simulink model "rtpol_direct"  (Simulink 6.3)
settings: Solver=ode45  SolverMode=SingleTasking  StartTime=0.0  StopTime=inf  FixedStep=h  RelTol=1e-3  AbsTol=1e-6
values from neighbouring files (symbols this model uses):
  adingain = [1.2*(pi*2/620/3)*[1 -1 -1 1 1 1] 1]    [hwinit.m]
  adinoffs = [-421 -511 -568 -518 -521 -410    0]    [hwinit.m]
  daoutgain = 127*[1 -1 -1 1 1 1 1]    [hwinit.m]
  daoutoffs = 127*[1 1 1 1 0.98 1 0]    [hwinit.m]
  h = 0.01    [design_pol.m]    (also in design_rot.m; design_wrist.m; rtrobot_init.m = 0.05; simpleregret.m = cfg.h)
  joint = [1 2 3 4 5]    [design_pol.m]    (also in design_rot.m = [1 5]; design_wrist.m = [5]; rtrobot_init.m = joint(:)+(0:6:6*(n-1))')
  Kd = [0.4 0.1 0.1]    [design_pol.m]    (also in design_rot.m = [0.3 0.1]; design_wrist.m = 0.01; mc_approx_vectorized.m = cfg.Kd)
  Ki = [0.6 0.3 0.9]/3    [design_pol.m]    (also in design_rot.m = [0.1 0.1]; design_wrist.m = 0)
  Kp = [0.5 0.2 1.0]    [design_pol.m]    (also in design_rot.m = [0.4 2]; design_wrist.m = 1.5)
undefined symbols (not defined in the file or in its folder): COM1, DiscIntNeverNeededParam, No
libraries: simulink x7, cstblocks x5, xpclib x4, rtlib x1

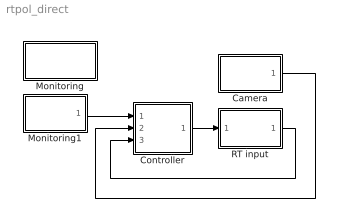
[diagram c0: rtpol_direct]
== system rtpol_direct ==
  Camera : Subsystem
  Controller : Subsystem
  Monitoring : Subsystem
  Monitoring1 : Subsystem
  RT input : Subsystem  InitFcn=rtclear all  mask{h=h, joint=joint, Port=COM1, laser=No, gripper=No}
      mask prompts: h "Sample time [s]:"; joint "Joints to control (e.g., [1 2 4])"; Port "Serial port:"; laser "Enable laser input"; gripper "Enable gripper current sensor"
      mask init:
      | hwinit;
      | sen = joint(:);                             % read joint angles
      | if strcmp(gripper,'Yes'),                   % if gripper current desired
      |     sen = [sen; 7];                         % add to the list
      | end;    
      |                                             
      | n = length(sen);                            % number of sensors to be read
      | sen = sen+(0:7:7*(n-1))';                   % convert into sequential index
      | sen_select = zeros(7,n);                    % prepare zeros
      | sen_select(sen) = 1;                        % assign 1 at the right places
      | 
      | act = joint(:);                             % control joint actuators
      | if strcmp(laser,'Yes'),                     % if laser desired
      |     act = [act; 7];                         % add to the list
      | end;    
      |                                             
      | n = length(act);                            % number of actuators to be controlled
      | act = act+(0:7:7*(n-1))';                   % convert into sequential index
      | act_select = zeros(7,n);                    % prepare zeros
      | act_select(act) = 1;                        % assign 1 at the right places
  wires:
  Camera/1(features) -> Controller/2(y)
  RT input/1(Angles) -> Controller/3(q)
  Monitoring1/1(r) -> Controller/1(r)
  Controller/1(out_2) -> RT input/1(Motors)

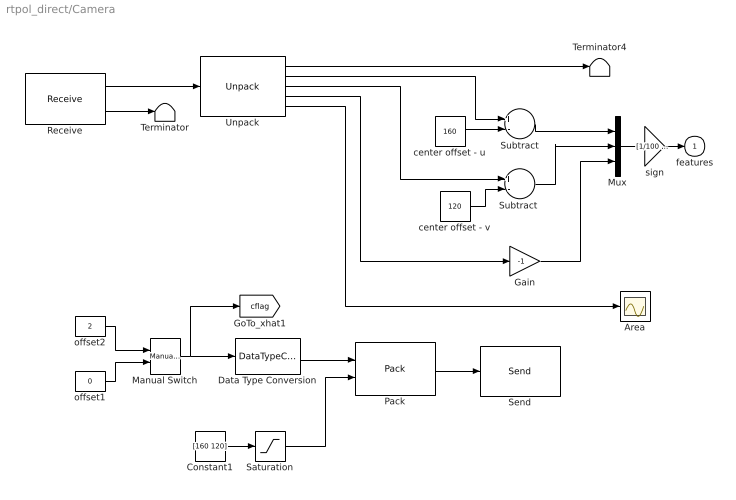
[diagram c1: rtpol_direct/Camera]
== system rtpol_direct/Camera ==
  Area : Scope
  Constant1 : Constant  Value=[160 120]
  Data Type Conversion : DataTypeConversion  OutDataTypeMode=uint8
  Gain : Gain  Gain=-1
  Manual Switch : simulink/Signal Routing/Manual Switch  sw=1  action=0
  Mux : Mux  Inputs=3
  Pack : xpclib/UDP/Pack  datatypes={'uint8','double'}  byteAlign=4
  Receive : xpclib/UDP/Receive  ipAddress=127.0.0.1  ipPort=6907  width=40  sampletime=h
  Saturation : Saturate  UpperLimit=[320 240]  LowerLimit=[0 0]
  Send : xpclib/UDP/Send  ipAddress=127.0.0.1  ipPort=6906  localPort=-1  sampletime=h
  Subtract : Sum  Inputs=+-  OutScaling=2^-10
  "Subtract " : Sum  Inputs=+-  OutScaling=2^-10
  Terminator : Terminator
  Terminator4 : Terminator
  Unpack : xpclib/UDP/Unpack  dimensions={1,1,1,1,1}  datatypes={'double','double','double','double','double'}  byteAlign=4
  center offset - u : Constant  Value=160
  center offset - v : Constant  Value=120
  offset1 : Constant  Value=0
  offset2 : Constant  Value=2
  sign : Gain  Gain=[1/100 1/100 1]  SampleTime=h
  features : Outport  InitialOutput=0
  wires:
  Receive/2 -> Terminator/1
  Receive/1 -> Unpack/1
  center offset - u/1 -> Subtract/2
  center offset - v/1 -> "Subtract "/2
  Unpack/2 -> Subtract/1
  Unpack/3 -> "Subtract "/1
  Unpack/4 -> Gain/1
  Subtract/1 -> Mux/1
  Unpack/5 -> Area/1
  Pack/1 -> Send/1
  Constant1/1 -> Saturation/1
  Data Type Conversion/1 -> Pack/1
  Saturation/1 -> Pack/2
  "Subtract "/1 -> Mux/2
  Manual Switch/1 -> Data Type Conversion/1, [cflag]
  offset2/1 -> Manual Switch/1
  offset1/1 -> Manual Switch/2
  Mux/1 -> sign/1
  Unpack/1 -> Terminator4/1
  sign/1 -> features/1
  Gain/1 -> Mux/3

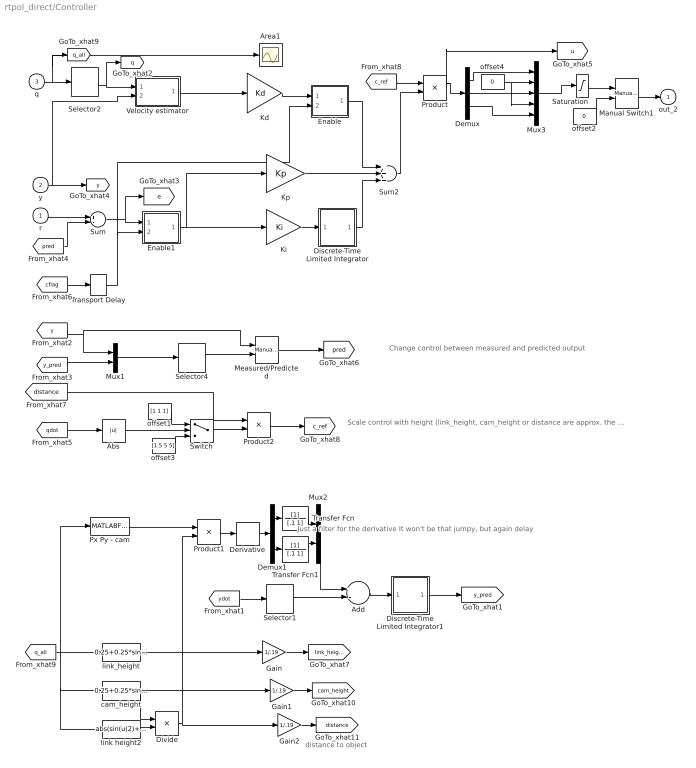
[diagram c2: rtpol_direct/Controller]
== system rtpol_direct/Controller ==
  note: Change control between measured and predicted output
  note: Scale control with height (link_height, cam_height or distance are approx. the same) and boost at low velocities
  note: distance to object
  note: Just a filter for the derivative It won't be that jumpy, but again delay
  r : Inport
  y : Inport  Port=2
  q : Inport  Port=3
  Abs : Abs
  Add : Sum  Inputs=+-  OutScaling=2^-10
  Area1 : Scope
  Demux : Demux  Outputs=3
  Demux1 : Demux  Outputs=2
  Derivative : Derivative
  Discrete-Time Limited Integrator : Subsystem  mask(Discrete-Time Limited Integrator.){}
      mask help: Discrete-Time Limited Integrator.
      mask init:
      | lower_limit=@1;upper_limit=@2;X0=@3;Ts=@4;
  Discrete-Time Limited Integrator1 : Subsystem  mask(Discrete-Time Limited Integrator.){}
      mask help: Discrete-Time Limited Integrator.
      mask init:
      | lower_limit=@1;upper_limit=@2;X0=@3;Ts=@4;
  Divide : Product  Inputs=*/  OutScaling=2^-10
  Enable : Subsystem
  Enable1 : Subsystem
  Gain : Gain  Gain=1/.19
  Gain1 : Gain  Gain=1/.19
  Gain2 : Gain  Gain=1/.19
  Kd : Gain  Gain=Kd  SampleTime=h
  Ki : Gain  Gain=Ki  SampleTime=h
  Kp : Gain  Gain=Kp  SampleTime=h
  Manual Switch1 : simulink/Signal Routing/Manual Switch  sw=1  action=0
  Measured/Predicted : simulink/Signal Routing/Manual Switch  sw=0  action=0
  Mux1 : Mux  Inputs=2
  Mux2 : Mux  Inputs=2
  Mux3 : Mux  Inputs=5
  Product : Product
  Product1 : Product
  Product2 : Product
  Px Py - cam : MATLABFcn  MATLABFcn=[0.25*cos(u(1))*cos(u(2))+0.25*cos(u(1))*cos(u(2)+u(3))-0.15*cos(u(1))*sin(u(2)+u(3)+u(4))-0.02*(cos(u(1))*cos(u(2)+u(3)+u(4))*sin(u(5))+sin(u(1))*cos(u(5))) 0.25*sin(u(1))*cos(u(2))+0.25*sin(u(1))*cos(u(2)+u(3))-0.15*sin(u(1))*cos(u(2)+u(3)+u(4))+0.02*(sin(u(1))*cos(u(2)+u(3)+u(4))*sin(u(5))+cos(u(1))*cos(u(5)))]
  Saturation : Saturate  UpperLimit=[0.6 inf 0.5 inf 1]  LowerLimit=[-0.6 -inf -0.5 -inf -1]
  Selector1 : Selector  Elements=[1 2]  InputPortWidth=3
  Selector2 : Selector  Elements=[1 3 5]  InputPortWidth=5
  Selector4 : Selector  Elements=[4 5 3]  InputPortWidth=5
  Sum : Sum  Inputs=+-  SampleTime=h
  Sum2 : Sum  Inputs=+++
  Switch : Switch  Threshold=[.005 0.01 0.001]
  Transfer Fcn : TransferFcn  Denominator=[.1 1]
  Transfer Fcn1 : TransferFcn  Denominator=[.1 1]
  Transport Delay : TransportDelay  DelayTime=.1
  Velocity estimator : Subsystem
  cam_height : Fcn  Expr=0.25+0.25*sin(u(2))+0.25*sin(u(2)+u(3))-0.15*cos(u(2)+u(3)+u(4))-0.02*sin(u(2)+u(3)+u(4))*sin(u(5))
  link height2 : Fcn  Expr=abs(sin(u(2)+u(3)+u(4)))
  link_height : Fcn  Expr=0.25+0.25*sin(u(2))+0.25*sin(u(2)+u(3))-0.15*cos(u(2)+u(3)+u(4))
  offset1 : Constant  Value=[1 1 1]
  offset2 : Constant  Value=0
  offset3 : Constant  Value=[1.5 5 5]
  offset4 : Constant  Value=0
  out_2 : Outport  InitialOutput=0
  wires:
  Discrete-Time Limited Integrator/1(out_1) -> Sum2/3
  Ki/1 -> Discrete-Time Limited Integrator/1(in_1)
  Enable1/1(Out) -> Ki/1, Kp/1
  Kp/1 -> Sum2/2
  r/1 -> Sum/1
  y/1 -> Velocity estimator/2(y), [y]
  Sum2/1 -> Product/2
  Velocity estimator/1(v) -> Kd/1
  q/1 -> Selector2/1, [q_all], Area1/1
  Sum/1 -> [e], Enable1/1(In1)
  Kd/1 -> Enable/1(In1)
  Enable/1(Out) -> Sum2/1
  [cflag] -> Transport Delay/1
  Transport Delay/1 -> Enable1/2(In2), Enable/2(In2)
  Selector2/1 -> Velocity estimator/1(q), [q]
  Product/1 -> [u], Demux/1
  Mux3/1 -> Saturation/1
  offset2/1 -> Manual Switch1/2
  Manual Switch1/1 -> out_2/1
  Saturation/1 -> Manual Switch1/1
  offset4/1 -> Mux3/2, Mux3/4
  Demux/1 -> Mux3/1
  Demux/2 -> Mux3/3
  Demux/3 -> Mux3/5
  Mux1/1 -> Selector4/1
  Selector4/1 -> Measured/Predicted/2
  [y_pred] -> Mux1/2
  [y] -> Mux1/1, Measured/Predicted/1
  Measured/Predicted/1 -> [pred]
  [pred] -> Sum/2
  [qdot] -> Abs/1
  Abs/1 -> Switch/2
  offset1/1 -> Switch/1
  offset3/1 -> Switch/3
  Switch/1 -> Product2/2
  [distance] -> Product2/1
  Product2/1 -> [c_ref]
  [c_ref] -> Product/1
  link_height/1 -> Gain/1
  Gain/1 -> [link_height]
  [ydot] -> Selector1/1
  Add/1 -> Discrete-Time Limited Integrator1/1(in_1)
  Discrete-Time Limited Integrator1/1(out_1) -> [y_pred]
  [q_all] -> link_height/1, cam_height/1, link height2/1, Px Py - cam/1
  cam_height/1 -> Divide/1, Gain1/1
  link height2/1 -> Divide/2
  Divide/1 -> Gain2/1, Product1/2
  Px Py - cam/1 -> Product1/1
  Product1/1 -> Derivative/1
  Derivative/1 -> Demux1/1
  Demux1/1 -> Transfer Fcn/1
  Mux2/1 -> Add/1
  Transfer Fcn1/1 -> Mux2/2
  Gain1/1 -> [cam_height]
  Gain2/1 -> [distance]
  Selector1/1 -> Add/2
  Transfer Fcn/1 -> Mux2/1
  Demux1/2 -> Transfer Fcn1/1

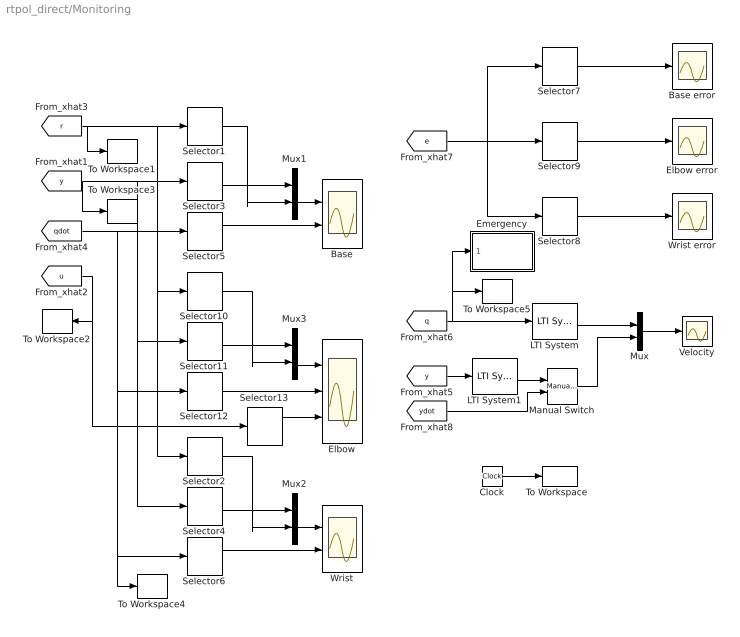
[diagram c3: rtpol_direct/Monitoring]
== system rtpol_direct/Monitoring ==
  Base : Scope  NumInputPorts=2
  Base error : Scope
  Clock : Clock
  Elbow : Scope  NumInputPorts=3
  Elbow error : Scope
  Emergency : Subsystem
  LTI System : cstblocks/LTI System  sys=Gder  IC=[]
  LTI System1 : cstblocks/LTI System  sys=Gder  IC=[]
  Manual Switch : simulink/Signal Routing/Manual Switch  sw=1  action=0
  Mux{,1..3} (4 alike) : Mux  Inputs=2
  Selector{1,3,5,7} (4 alike) : Selector  InputPortWidth=ny
  Selector{10..13} (4 alike) : Selector  Elements=2  InputPortWidth=ny
  Selector{2,4,6,8..9} (5 alike) : Selector  Elements=3  InputPortWidth=ny
  "To Workspace  " : ToWorkspace  VariableName=t  SampleTime=h  SaveFormat=Array
  To Workspace1 : ToWorkspace  VariableName=r  SampleTime=h  SaveFormat=Array
  To Workspace2 : ToWorkspace  VariableName=u  SampleTime=h  SaveFormat=Array
  To Workspace3 : ToWorkspace  VariableName=y  SampleTime=h  SaveFormat=Array
  To Workspace4 : ToWorkspace  VariableName=qdot  SampleTime=h  SaveFormat=Array
  To Workspace5 : ToWorkspace  VariableName=q  SampleTime=h  SaveFormat=Array
  Velocity : Scope
  Wrist : Scope  NumInputPorts=2
  Wrist error : Scope
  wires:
  Selector6/1 -> Wrist/2
  [u] -> To Workspace2/1, Selector13/1
  [y] -> To Workspace3/1, Selector3/1, Selector4/1, Selector11/1
  Mux1/1 -> Base/1
  [r] -> To Workspace1/1, Selector1/1, Selector2/1, Selector10/1
  Clock/1 -> "To Workspace  "/1
  Mux2/1 -> Wrist/1
  Selector1/1 -> Mux1/2
  Selector2/1 -> Mux2/2
  Selector3/1 -> Mux1/1
  Selector4/1 -> Mux2/1
  [qdot] -> Selector5/1, Selector6/1, To Workspace4/1, Selector12/1
  Selector5/1 -> Base/2
  Mux/1 -> Velocity/1
  LTI System/1 -> Mux/1
  [y] -> LTI System1/1
  [q] -> LTI System/1, To Workspace5/1, Emergency/1(In1)
  Selector8/1 -> Wrist error/1
  [e] -> Selector7/1, Selector8/1, Selector9/1
  Selector7/1 -> Base error/1
  Selector9/1 -> Elbow error/1
  Selector12/1 -> Elbow/2
  Mux3/1 -> Elbow/1
  Selector10/1 -> Mux3/2
  Selector11/1 -> Mux3/1
  LTI System1/1 -> Manual Switch/1
  [ydot] -> Manual Switch/2
  Manual Switch/1 -> Mux/2
  Selector13/1 -> Elbow/3

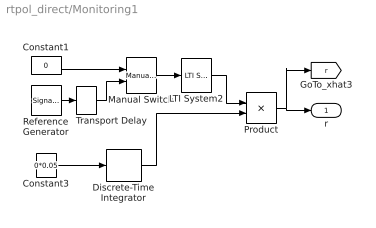
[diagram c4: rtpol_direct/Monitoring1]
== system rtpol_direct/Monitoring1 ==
  Constant1 : Constant  Value=0
  Constant3 : Constant  Value=0*0.05
  Discrete-Time Integrator : DiscreteIntegrator  InitialCondition=1  SampleTime=5  ICPrevOutput=DiscIntNeverNeededParam  ICPrevScaledInput=DiscIntNeverNeededParam
  LTI System2 : cstblocks/LTI System  sys=Fref  IC=[]
  Manual Switch : simulink/Signal Routing/Manual Switch  sw=1  action=0
  Product : Product
  Reference Generator : SignalGenerator  WaveForm=square  Amplitude=[0.4*0 0 0.4]  Frequency=1/5
  Transport Delay : TransportDelay  DelayTime=.5
  r : Outport
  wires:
  Product/1 -> r/1, [r]
  Constant3/1 -> Discrete-Time Integrator/1
  Discrete-Time Integrator/1 -> Product/2
  Manual Switch/1 -> LTI System2/1
  Reference Generator/1 -> Transport Delay/1
  Constant1/1 -> Manual Switch/1
  Transport Delay/1 -> Manual Switch/2
  LTI System2/1 -> Product/1

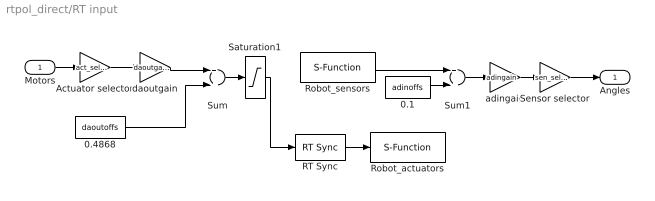
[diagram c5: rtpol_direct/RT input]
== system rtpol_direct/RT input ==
  Motors : Inport
  0.1 : Constant  Value=adinoffs
  0.4868 : Constant  Value=daoutoffs
  Actuator selector : Gain  Gain=act_select  Multiplication=Matrix(K*u)
  RT Sync : rtlib/RT Sync
  Robot_actuators : S-Function  FunctionName=sfserialout  Parameters=Ts, com  mask(Serial Out){Ts=h, Port=Port}
      mask prompts: Ts "Sample time:"; Port "Serial port:"
      mask help: Serial line output block
      mask init:
      | com = xserial('Port',Port,'Baudrate',115200);
  Robot_sensors : S-Function  FunctionName=sfserialin  Parameters=Ts, com  mask(Serial Out){Ts=h, Port=Port}
      mask prompts: Ts "Sample time:"; Port "Serial port:"
      mask help: Serial line output block
      mask init:
      | com = xserial('Port',Port,'Baudrate',115200);
  Saturation1 : Saturate  UpperLimit=255  LowerLimit=0
  Sensor selector : Gain  Gain=sen_select'  Multiplication=Matrix(K*u)
  Sum : Sum
  Sum1 : Sum
  adingain : Gain  Gain=adingain
  daoutgain : Gain  Gain=daoutgain
  Angles : Outport
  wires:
  RT Sync/1 -> Robot_actuators/1
  Actuator selector/1 -> daoutgain/1
  Sensor selector/1 -> Angles/1
  Saturation1/1 -> RT Sync/1
  daoutgain/1 -> Sum/1
  adingain/1 -> Sensor selector/1
  Robot_sensors/1 -> Sum1/1
  0.1/1 -> Sum1/2
  Sum1/1 -> adingain/1
  Motors/1 -> Actuator selector/1
  0.4868/1 -> Sum/2
  Sum/1 -> Saturation1/1

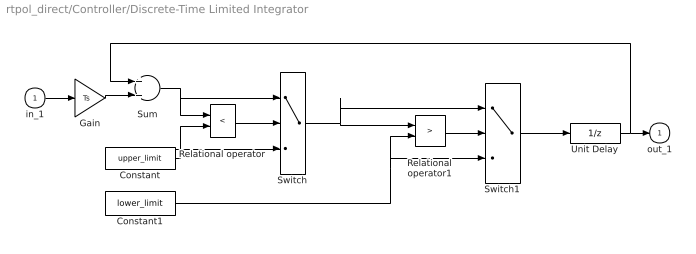
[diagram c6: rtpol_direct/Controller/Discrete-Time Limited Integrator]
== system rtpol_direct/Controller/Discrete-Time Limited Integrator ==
  in_1 : Inport
  Constant : Constant  Value=upper_limit
  Constant1 : Constant  Value=lower_limit
  Gain : Gain  Gain=Ts
  Relational operator : RelationalOperator  Operator=<
  Relational operator1 : RelationalOperator  Operator=>
  Sum : Sum
  Switch : Switch  Threshold=0.5
  Switch1 : Switch  Threshold=0.5
  Unit Delay : UnitDelay  X0=X0  SampleTime=Ts
  out_1 : Outport  InitialOutput=0
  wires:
  in_1/1 -> Gain/1
  Relational operator/1 -> Switch/2
  Sum/1 -> Relational operator/1, Switch/1
  Gain/1 -> Sum/2
  Constant/1 -> Relational operator/2, Switch/3
  Switch/1 -> Switch1/1, Relational operator1/1
  Relational operator1/1 -> Switch1/2
  Constant1/1 -> Switch1/3, Relational operator1/2
  Switch1/1 -> Unit Delay/1
  Unit Delay/1 -> Sum/1, out_1/1

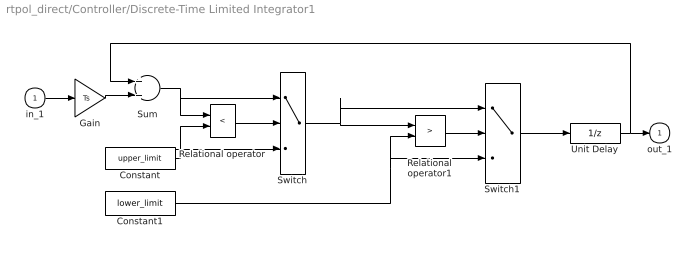
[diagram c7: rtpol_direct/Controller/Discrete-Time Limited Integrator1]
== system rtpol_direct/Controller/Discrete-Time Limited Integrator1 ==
  in_1 : Inport
  Constant : Constant  Value=upper_limit
  Constant1 : Constant  Value=lower_limit
  Gain : Gain  Gain=Ts
  Relational operator : RelationalOperator  Operator=<
  Relational operator1 : RelationalOperator  Operator=>
  Sum : Sum
  Switch : Switch  Threshold=0.5
  Switch1 : Switch  Threshold=0.5
  Unit Delay : UnitDelay  X0=X0  SampleTime=Ts
  out_1 : Outport  InitialOutput=0
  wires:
  in_1/1 -> Gain/1
  Relational operator/1 -> Switch/2
  Sum/1 -> Relational operator/1, Switch/1
  Gain/1 -> Sum/2
  Constant/1 -> Relational operator/2, Switch/3
  Switch/1 -> Switch1/1, Relational operator1/1
  Relational operator1/1 -> Switch1/2
  Constant1/1 -> Switch1/3, Relational operator1/2
  Switch1/1 -> Unit Delay/1
  Unit Delay/1 -> Sum/1, out_1/1

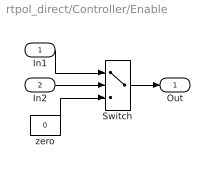
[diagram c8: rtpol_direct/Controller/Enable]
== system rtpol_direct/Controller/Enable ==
  In1 : Inport
  In2 : Inport  Port=2
  Switch : Switch  Threshold=0.5
  zero : Constant  Value=0
  Out : Outport
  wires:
  zero/1 -> Switch/3
  In2/1 -> Switch/2
  In1/1 -> Switch/1
  Switch/1 -> Out/1

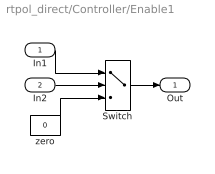
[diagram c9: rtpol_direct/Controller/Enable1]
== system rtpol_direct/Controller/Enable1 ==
  In1 : Inport
  In2 : Inport  Port=2
  Switch : Switch  Threshold=0.5
  zero : Constant  Value=0
  Out : Outport
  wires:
  zero/1 -> Switch/3
  In2/1 -> Switch/2
  In1/1 -> Switch/1
  Switch/1 -> Out/1

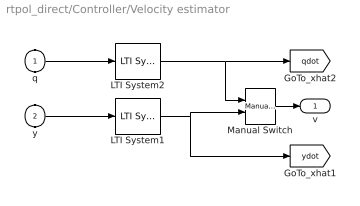
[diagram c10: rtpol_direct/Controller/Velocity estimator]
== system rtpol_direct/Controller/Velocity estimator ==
  q : Inport
  y : Inport  Port=2
  LTI System1 : cstblocks/LTI System  sys=Gder  IC=[]
  LTI System2 : cstblocks/LTI System  sys=Gder1  IC=[]
  Manual Switch : simulink/Signal Routing/Manual Switch  sw=1  action=0
  v : Outport
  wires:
  LTI System2/1 -> Manual Switch/1, [qdot]
  LTI System1/1 -> Manual Switch/2, [ydot]
  y/1 -> LTI System1/1
  q/1 -> LTI System2/1
  Manual Switch/1 -> v/1

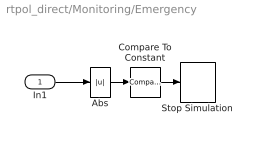
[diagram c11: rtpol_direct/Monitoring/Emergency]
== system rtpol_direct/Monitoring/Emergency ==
  In1 : Inport
  Abs : Abs
  Compare To Constant : simulink/Logic and Bit Operations/Compare To Constant  relop=>  const=[0.6 0.5 0.9]  LogicOutDataTypeMode=boolean  ZeroCross=off
  Stop Simulation : Stop
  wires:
  Abs/1 -> Compare To Constant/1
  Compare To Constant/1 -> Stop Simulation/1
  In1/1 -> Abs/1
